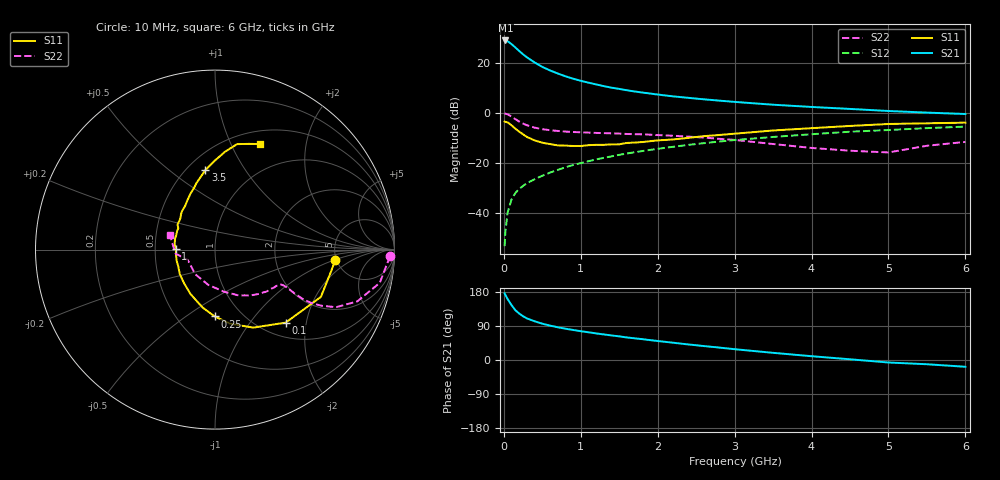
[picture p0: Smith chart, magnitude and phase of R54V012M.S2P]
! SIEMENS Small Signal Semiconductors
! BFR183
! Si NPN RF Bipolar Junction Transistor in SOT23
! VCE = 4 V  IC = 12 mA
! Common Emitter S-Parameters:  May  1996
# GHz  S  MA  R  50
!  f  S11  S21  S12  S22
! GHz  MAG  ANG  MAG  ANG  MAG  ANG  MAG  ANG
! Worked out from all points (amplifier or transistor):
!   36 points, 10 MHz to 6 GHz, reference 50 ohm
!   highest |S21| = 28.9 dB at 20 MHz (marker M1)
!   |S21| within 3 dB of that: start of sweep to 157.1 MHz
!   unconditionally stable (mu >= 1): 719.1 MHz to 2.462 GHz
!   at 250 MHz: K = 0.67, MSG = 26.2 dB, |S12| = -29.1 dB
!   at 1.4 GHz: K = 1.05, MAG = 12.3 dB, |S12| = -17.3 dB
!   at 6 GHz: K = 0.89, MSG = 2.5 dB, |S12| = -5.5 dB
!   S11 on the Smith chart (normalised r, x): 10 MHz: 4.85, -1.06; 100 MHz: 1.27, -1.52; 250 MHz: 0.75, -0.65; 1 GHz: 0.64, +0.01; 3.5 GHz: 0.61, +0.68; 6 GHz: 0.65, +1.29
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0.01  0.6716 -5.1  27.73 175.9  0.0022 88.8  0.9761 -2.2
0.02  0.6595 -10.0  27.77 171.7  0.0043 87.3  0.962 -4.7
0.05  0.6461 -24.1  26.72 160.6  0.0104 78.6  0.9365 -11.4
0.1  0.5659 -46.0  23.48 144.7  0.0189 72.4  0.8434 -20.0
0.15  0.484 -63.9  20.11 131.4  0.0253 67.1  0.7479 -25.4
0.2  0.4222 -78.2  17.12 122.5  0.0306 65.3  0.6711 -27.8
0.25  0.3725 -90.2  14.68 115.4  0.035 63.8  0.6112 -29.0
0.3  0.3308 -101.9  12.8 109.7  0.0396 64.8  0.5664 -29.4
0.4  0.2826 -118.9  10.12 102.2  0.0474 65.0  0.5074 -28.9
0.5  0.2539 -133.0  8.248 95.8  0.0558 66.1  0.4732 -28.2
0.6  0.2389 -145.3  7.018 90.8  0.0643 66.8  0.4512 -27.8
0.7  0.2246 -156.1  6.1 86.4  0.0729 67.2  0.4364 -27.6
0.8  0.2224 -164.6  5.364 82.6  0.0821 67.0  0.4241 -27.7
1  0.2182 178.4  4.359 76.0  0.0995 67.0  0.4104 -28.5
1.1  0.2268 172.6  4 73.2  0.1086 66.7  0.4047 -29.7
1.3  0.2304 159.6  3.414 67.5  0.127 65.7  0.3944 -31.3
1.6  0.2514 146.1  2.82 59.5  0.1549 63.7  0.3794 -35.1
2.2  0.295 124.4  2.133 45.6  0.2107 58.4  0.35 -44.6
3.5  0.4456 97.0  1.454 18.9  0.331 43.3  0.2393 -78.2
4.5  0.5486 84.1  1.198 1.9  0.421 30.9  0.1759 -128.8
5.5  0.6194 72.0  1.012 -11.2  0.4963 19.1  0.2209 -174.3
6  0.6383 67.1  0.949 -17.9  0.5319 11.5  0.2637 162.4
